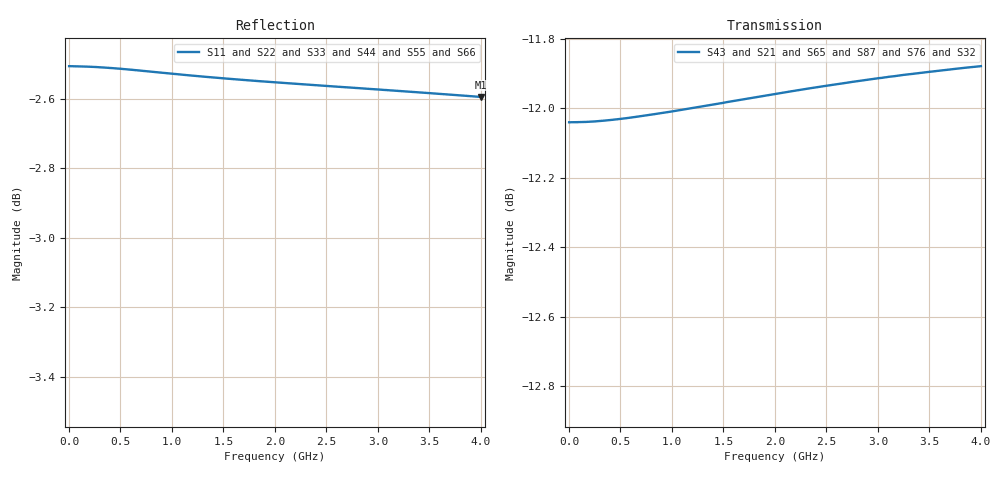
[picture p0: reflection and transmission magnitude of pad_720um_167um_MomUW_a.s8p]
! Created Thu Sep 17 15:57:33 2015
# ghz S ma R 50
! 8 Port Network Data from data block
! freq  magS11  angS11  magS12  angS12  magS13  angS13  magS14  angS14
!  magS15  angS15  magS16  angS16  magS17  angS17  magS18  angS18
!  magS21  angS21  magS22  angS22  magS23  angS23  magS24  angS24
!  magS25  angS25  magS26  angS26  magS27  angS27  magS28  angS28
!  magS31  angS31  magS32  angS32  magS33  angS33  magS34  angS34
!  magS35  angS35  magS36  angS36  magS37  angS37  magS38  angS38
!  magS41  angS41  magS42  angS42  magS43  angS43  magS44  angS44
!  magS45  angS45  magS46  angS46  magS47  angS47  magS48  angS48
!  magS51  angS51  magS52  angS52  magS53  angS53  magS54  angS54
!  magS55  angS55  magS56  angS56  magS57  angS57  magS58  angS58
!  magS61  angS61  magS62  angS62  magS63  angS63  magS64  angS64
!  magS65  angS65  magS66  angS66  magS67  angS67  magS68  angS68
!  magS71  angS71  magS72  angS72  magS73  angS73  magS74  angS74
!  magS75  angS75  magS76  angS76  magS77  angS77  magS78  angS78
!  magS81  angS81  magS82  angS82  magS83  angS83  magS84  angS84
!  magS85  angS85  magS86  angS86  magS87  angS87  magS88  angS88
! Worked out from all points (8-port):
!   46 points, 1 MHz to 4 GHz, reference 50 ohm
!   strongest paths, dB at 1 MHz, 1.001 GHz, 2.001 GHz, 3.063 GHz, 4 GHz:
!     S43: -12.0, -12.0, -12.0, -11.9, -11.9
!     S21: -12.0, -12.0, -12.0, -11.9, -11.9
!     S65: -12.0, -12.0, -12.0, -12.0, -11.9
!     S87: -12.0, -12.0, -12.0, -12.0, -11.9
!     S76: -12.0, -12.0, -12.0, -12.0, -12.0
!     S32: -12.0, -12.0, -12.0, -12.0, -12.0
!   lowest |S11| = -2.6 dB at 4 GHz (marker M1), VSWR 6.75, Z = 7.41 + j0.00323 ohm
!   |S11| at or under -10 dB: nowhere
